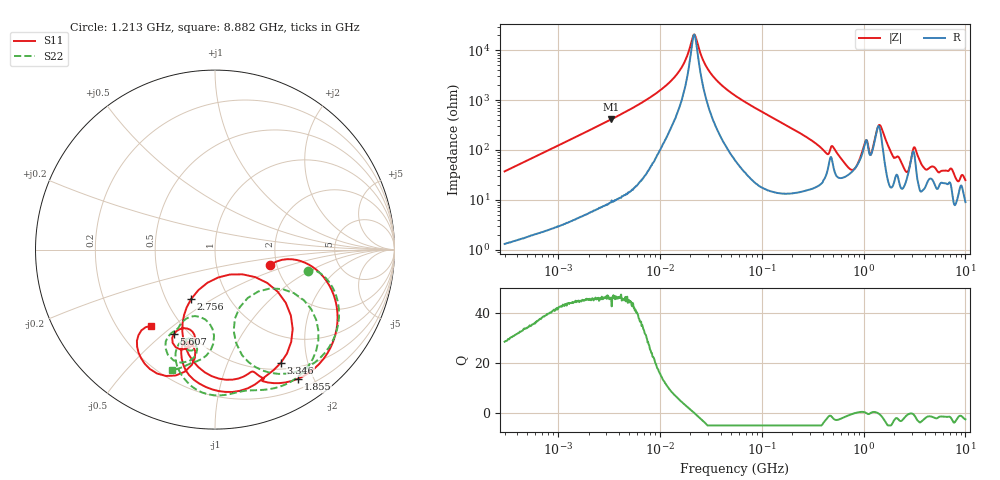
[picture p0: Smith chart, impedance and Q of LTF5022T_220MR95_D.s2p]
! S-Parameter Data Generated by TDK Corporation
! Copyright(C) 2020 TDK Corporation.
! All Rights Reserved.
! TDK P/N: LTF5022T-220MR95-D (Inductor)
! Property: L=22uH at 100kHz
! Size(LxWxT): 6.5x5x2.2mm
! Model Type: s2p (Touchstone File Format Version 1.0)
! Frequency: DC=Yes Start=0.3MHz Stop=10000MHz 802points Log-sweep
! Model Generated on Apr. 23, 2020
! Port Assignments:
!  1 ---@@@--- 2
! Applicable Conditions:
!  Temperature = 25 degC
!  DC Bias Current = 0 A
!  Small Signal Operation
! Terms and conditions regarding TDK Simulation Models
! (1)This simulation model is being provided solely for informational purposes. Please refer to the specifications of the products in terms of detailed characteristics of such products.
! (2)In no event shall TDK Corporation of any of its subsidiaries be liable for any loss or damage arising, directly or indirectly,
!  From any information contained in this simulation model, including, but not limited to loss or damages arising from any inaccuracies, omissions or errors in connection with such information.
! (3)Any and all copyrights on this simulation model are owned by TDK Corporation.
!  Duplication or redistribution of this simulation model without prior written permission from TDK Corporation is prohibited.
! (4)This simulation model is subject to any modification or change without any prior notice.
! (5)Neither TDK Corporation nor any of its subsidiaries shall make any warranty, express or implied,
!  Including but not limited to the correctness, implied warranties of merchantability and fitness for a particular purpose with respect to this simulation models.
! (6)The use of this simulation model shall be deemed to have consented to the terms and conditions hereof.
# Hz S MA R 50
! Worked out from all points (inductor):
!   801 points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, 300 kHz to 10 GHz, reference 50 ohm
!   read as 1/Y11, port 2 shorted: L = 19.6 uH near 318.3 kHz
!   highest Q = 46.7 at 3.33 MHz (marker M1), where L = 19.6 uH
!   self-resonance near 21.58 MHz
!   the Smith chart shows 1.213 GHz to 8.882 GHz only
!   S11 on the Smith chart (normalised r, x): 1.213 GHz: 1.85, -0.35; 1.855 GHz: 0.33, -1.78; 2.756 GHz: 0.67, -0.40; 3.346 GHz: 0.58, -1.58; 5.607 GHz: 0.42, -0.54; 8.882 GHz: 0.34, -0.42
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300000  0.3444 67.9  0.927 -20.1  0.9267 -20.1  0.3441 67.9
1713600  0.8935 25.4  0.4296 -63.3  0.4297 -63.3  0.8934 25.4
3330145  0.9662 13.6  0.2377 -75.1  0.2377 -75.1  0.9661 13.6
9671944  0.9935 3.9  0.07257 -83.1  0.07257 -83.1  0.9934 3.9
1.80882e7  0.9949 0.8  0.02418 -77.8  0.02419 -77.8  0.9948 0.8
2.630692e7  0.9953 -0.8  0.004568 -2.0  0.004568 -2.2  0.9953 -0.8
5.477226e7  0.9947 -4.6  0.05088 80.9  0.05086 80.9  0.9946 -4.6
3.126428e8  0.8649 -33.2  0.3916 49.4  0.3916 49.4  0.8696 -32.5
5.285151e8  0.6691 -39.0  0.531 25.0  0.5308 25.0  0.6715 -52.1
8.758105e8  0.3558 -31.0  0.6967 -25.7  0.6965 -25.7  0.2184 -29.6
1.212691e9  0.3205 -15.3  0.5626 -48.0  0.5628 -47.9  0.5299 -13.1
1.767019e9  0.8618 -47.6  0.1562 -100.4  0.1562 -100.3  0.8393 -48.6
1.854885e9  0.8553 -57.3  0.1168 -62.9  0.1169 -62.9  0.7978 -60.0
2.23379e9  0.7191 -75.6  0.3063 -88.5  0.3065 -88.6  0.4358 -30.3
2.477118e9  0.6624 -97.9  0.1123 -73.9  0.112 -73.8  0.8176 -48.3
2.756092e9  0.3055 -115.8  0.2592 -60.2  0.2603 -60.0  0.8275 -70.7
3.34571e9  0.7299 -59.8  0.08008 -97.0  0.08239 -99.8  0.7869 -97.5
4.457691e9  0.5767 -108.7  0.3385 -94.3  0.3363 -94.4  0.5522 -107.8
5.607117e9  0.5225 -116.0  0.2014 -137.6  0.2009 -137.9  0.6124 -116.8
7.06055e9  0.5527 -102.5  0.06394 -155.3  0.06155 -159.9  0.3932 -97.8
8.881947e9  0.5554 -130.1  0.1701 113.9  0.1673 114.2  0.7135 -109.4
1e10  0.7425 -129.3  0.03253 20.4  0.03215 20.3  0.843 -118.6
